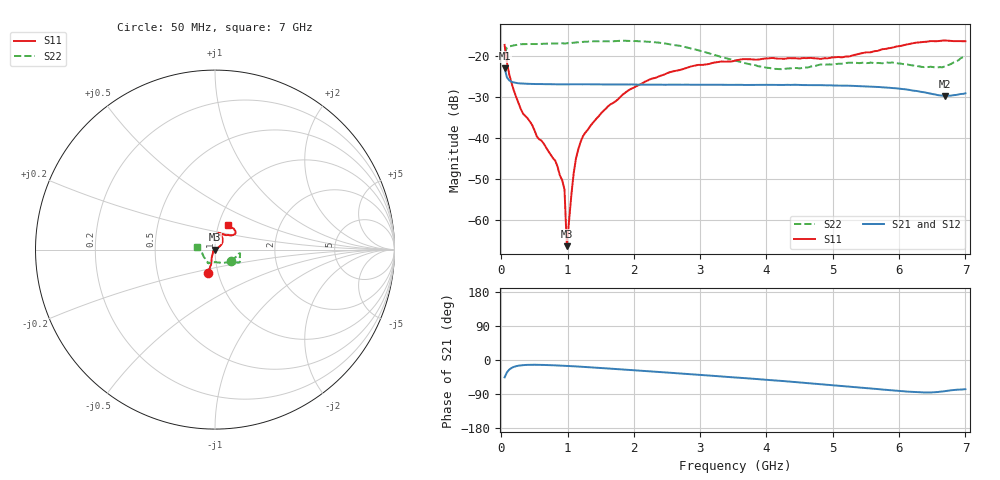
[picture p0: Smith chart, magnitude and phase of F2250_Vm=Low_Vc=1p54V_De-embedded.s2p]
! Integrated Device Technology
! Corporate Headquarters
! 6024 Silver Creek Valley Road
! San Jose, CA 95138  USA
! Phone:  1-408-284-8200
! Toll Free:  1-800-223-1366
! Webpage:  http://www.idt.com/
! Timing and RF Division
! 515 Groton Road, Suite 102
! Westford, MA 01886-6024
! Device:  F2250
! Description: Voltage Variable RF Attenuator
! Frequency:  50.0 -  6000.00 MHz
! Package:  3x3 mm Thin QFN Plastic Package: 16 pin
! Ports:  2 RF, 3 DC
!  Pin  1  = GND
!  Pin  2  = NC
!  Pin  3  = RF1  = Port 1
!  Pin  4  = NC
!  Pin  5  = GND
!  Pin  6  = GND
!  Pin  7  = GND
!  Pin  8  = GND
!  Pin  9  = NC
!  Pin 10  = RF2  = Port 2
!  Pin 11  = NC
!  Pin 12  = GND
!  Pin 13  = GND
!  Pin 14  = VCNTRL
!  Pin 15  = VDD
!  Pin 16  = VMODE
! Vcntrl:  1.540 Volts
! Vmode:  +0.000 Volts
! Vdd:  +3.30  Volts
! Current:  1.188 mA
! Data:  The device was measured on a the F2250 evaluation board which has
!  individual transmission lines to the RF pins.  Data was collected
!  using a calibrated network analyzer.  The evaluation board was
!  de-embedded using a TRL calibration technique.
!  The reference plane is the edge of the package pin.
! Misc:  SN 10
!  Action Tracker AT0258
! Date Measured:  2014-11-26
! Date:  2015-10-15  MJV
! Note:
!  Integrated Device Technology supplies this data as a sample of measured
!  data at the package pin for this product.  Your particular data for this
!  product may vary.
!  Data was taken at 25 degrees C.
!  Integrated Device Technology reserves the right to change this data at anytime.
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# GHz S dB R 50
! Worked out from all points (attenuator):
!   201 points, 50 MHz to 7 GHz, reference 50 ohm
!   highest |S21| = -22.88 dB at 50 MHz (marker M1); lowest = -29.6 dB at 6.687 GHz (marker M2)
!   lowest |S11| = -66.3 dB at 988.2 MHz (marker M3), VSWR 1.00, Z = 50 + j0.0204 ohm
!   |S11| at or under -10 dB: start of sweep to end of sweep
!   |S22| runs from -23.1 to -16.2 dB; largest |S21 - S12| = 0.00028
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0.05  -17.19 -106.7  -22.88 -45.8  -22.87 -45.8  -19.43 -35.6
0.1195  -24.32 -108.4  -25.85 -25.3  -25.85 -25.3  -17.59 -11.6
0.29325  -32.80 -119.9  -26.59 -14.2  -26.58 -14.1  -17.02 -9.0
0.467  -36.77 -137.5  -26.70 -12.6  -26.73 -12.6  -16.98 -9.3
0.5365  -39.54 -143.9  -26.74 -12.7  -26.73 -12.7  -16.98 -10.6
0.8145  -45.46 178.5  -26.80 -14.2  -26.80 -14.2  -16.85 -15.1
0.91875  -50.21 152.8  -26.81 -15.0  -26.81 -15.0  -16.78 -17.1
0.9535  -52.48 -176.8  -26.81 -15.3  -26.79 -15.3  -16.85 -17.4
0.98825  -66.28 155.2  -26.78 -15.6  -26.79 -15.6  -16.79 -17.7
1.0925  -48.41 27.7  -26.80 -16.5  -26.78 -16.5  -16.66 -18.8
1.12725  -44.80 27.6  -26.79 -16.9  -26.79 -16.9  -16.59 -19.4
1.2315  -39.47 26.3  -26.80 -18.0  -26.79 -18.0  -16.44 -21.1
1.5095  -33.79 30.9  -26.82 -21.3  -26.80 -21.3  -16.33 -23.3
1.82225  -29.43 33.9  -26.84 -24.9  -26.83 -24.9  -16.18 -25.9
2.37825  -24.86 43.9  -26.87 -31.6  -26.89 -31.6  -16.63 -29.5
2.93425  -22.18 57.6  -26.91 -38.5  -26.92 -38.4  -18.33 -35.8
3.525  -21.04 70.9  -26.94 -46.0  -26.94 -46.0  -21.00 -55.3
4.11575  -20.41 78.7  -26.95 -53.8  -26.93 -53.8  -23.05 -84.3
4.7065  -20.45 71.5  -26.97 -62.2  -26.97 -62.2  -22.36 -108.3
5.85325  -17.98 39.5  -27.64 -79.6  -27.63 -79.6  -21.55 -118.6
6.68725  -16.11 48.2  -29.63 -82.3  -29.62 -82.3  -22.45 -167.3
7  -16.29 62.8  -29.00 -77.1  -29.03 -77.0  -19.88 170.6
